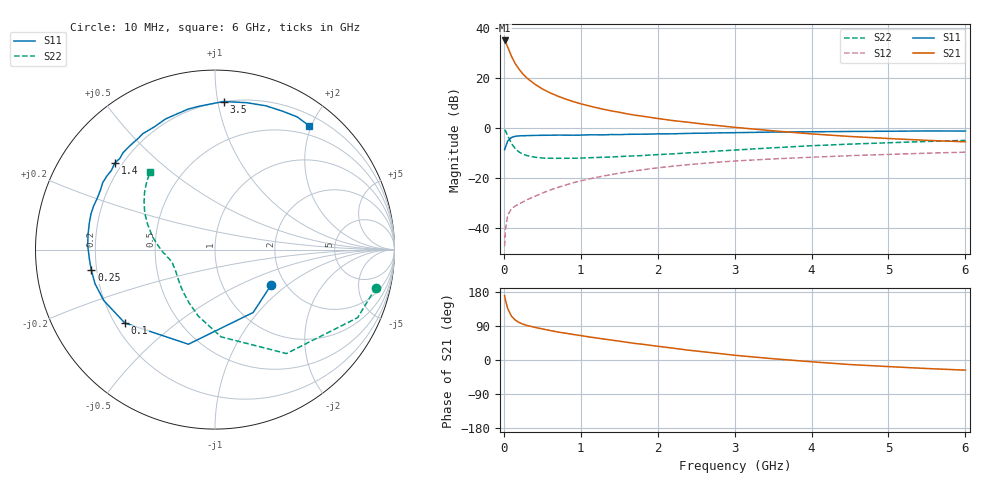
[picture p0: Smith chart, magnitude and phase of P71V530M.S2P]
! SIEMENS Small Signal Semiconductors
! BFP196
! Si NPN RF Bipolar Junction Transistor in SOT143
! VCE = 1.5 V  IC = 30 mA
! Common Emitter S-Parameters:  May  1996
# GHz  S  MA  R  50
!  f  S11  S21  S12  S22
! GHz  MAG  ANG  MAG  ANG  MAG  ANG  MAG  ANG
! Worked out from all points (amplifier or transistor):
!   36 points, 10 MHz to 6 GHz, reference 50 ohm
!   highest |S21| = 34.9 dB at 10 MHz (marker M1)
!   |S21| within 3 dB of that: start of sweep to 55.59 MHz
!   unconditionally stable (mu >= 1): 534.1 MHz to 4.385 GHz
!   at 250 MHz: K = 0.74, MSG = 25.4 dB, |S12| = -29.5 dB
!   at 1.4 GHz: K = 1.10, MAG = 10.8 dB, |S12| = -18.6 dB
!   at 6 GHz: K = 0.99, MSG = 2.1 dB, |S12| = -9.7 dB
!   S11 on the Smith chart (normalised r, x): 10 MHz: 1.69, -0.77; 100 MHz: 0.24, -0.34; 250 MHz: 0.18, -0.08; 1.4 GHz: 0.17, +0.36; 3.5 GHz: 0.20, +1.04; 6 GHz: 0.35, +1.96
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0.01  0.3695 -32.1  55.31 169.7  0.0044 80.2  0.9213 -13.3
0.02  0.4098 -58.7  52.31 158.7  0.0093 71.6  0.8805 -25.5
0.05  0.5477 -105.7  41.1 135.9  0.0182 55.0  0.7028 -55.5
0.1  0.6479 -140.9  26.65 115.4  0.0247 44.4  0.4873 -86.0
0.15  0.6817 -155.4  18.92 105.1  0.0279 43.5  0.3824 -104.0
0.2  0.695 -164.1  14.61 98.8  0.0307 44.3  0.329 -116.3
0.25  0.6984 -170.6  11.76 94.5  0.0336 46.8  0.2978 -125.8
0.3  0.7014 -175.0  9.865 91.2  0.037 48.6  0.2811 -132.5
0.4  0.7098 178.1  7.49 86.3  0.0432 52.1  0.261 -142.4
0.5  0.7124 173.2  5.993 82.0  0.0502 54.7  0.2516 -149.0
0.6  0.7155 168.2  5.005 77.9  0.0576 56.3  0.2484 -153.6
0.7  0.7192 163.9  4.306 73.9  0.0649 57.1  0.248 -157.0
0.9  0.7157 156.4  3.353 67.5  0.0807 57.3  0.2483 -162.1
1.1  0.7283 149.3  2.763 61.1  0.0954 56.5  0.2541 -165.5
1.4  0.738 139.1  2.18 52.6  0.1176 53.7  0.2637 -169.8
1.7  0.7475 129.9  1.8 43.8  0.1393 50.7  0.2765 -174.2
2.2  0.7628 116.3  1.399 31.2  0.173 43.9  0.3041 179.3
2.8  0.7969 100.8  1.106 17.1  0.2084 35.7  0.3476 169.8
3.5  0.8264 86.7  0.875 3.4  0.2411 26.1  0.4017 159.3
4.5  0.8498 70.5  0.675 -12.0  0.2798 14.3  0.4756 146.2
5.5  0.8698 58.2  0.565 -22.5  0.3136 3.6  0.5371 135.1
6  0.8666 52.8  0.528 -26.8  0.3285 -2.2  0.5646 129.6
